(* Logix 5000 AddOnInstructionDefinition export SPEL_Above; software revision 30.01; part 7 of 9 *)

ADD_ON_INSTRUCTION SPEL_PointCoordGet   (* revision 1.2, vendor SEIKO EPSON CORP. *)
// Acquires the coordinate of the specified point.
VAR_OUTPUT
   InCycle : BOOL; {access Read Only, visible}
   Done : BOOL; {access Read Only, visible}
   Error : BOOL; {access Read Only, visible}
END_VAR
VAR_INPUT
   Start : BOOL; {access None, required}
   Point : INT; {access None, required}
   AxisNum : INT; {access None, required}
END_VAR
VAR_OUTPUT
   Value : REAL; {access Read Only, visible}
END_VAR
VAR_IN_OUT
   ExtInputs : AB:ETHERNET_MODULE_INT_128Bytes:I:0; {required}
   ExtOutputs : AB:ETHERNET_MODULE_INT_128Bytes:O:0; {required}
END_VAR
VAR_INPUT
   ErrCode1 : INT; {access None, visible}
   ErrCode2 : INT; {access None, visible}
END_VAR
VAR
   OneShotStart : BOOL; {access None}
   StartInit : BOOL; {access None}
   ExecGetPointCoord : SPEL_ExecCmd := (MaxTime := 3000); {access None}
   Coordinate_INTS : INT[2]; {access None}
   Coordinatex1000 : DINT; {access None}
END_VAR

ROUTINE Logic   (* ladder *)
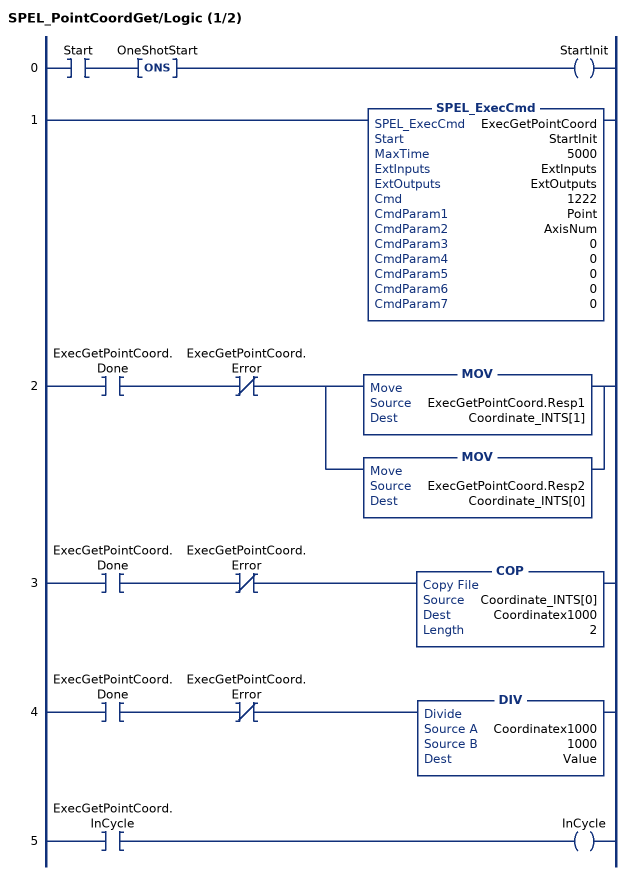
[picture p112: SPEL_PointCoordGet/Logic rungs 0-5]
   0: XIC(Start)ONS(OneShotStart)OTE(StartInit);
   1: SPEL_ExecCmd(ExecGetPointCoord,StartInit,5000,ExtInputs,ExtOutputs,1222,Point,AxisNum,0,0,0,0,0);
   2: XIC(ExecGetPointCoord.Done)XIO(ExecGetPointCoord.Error)[MOV(ExecGetPointCoord.Resp1,Coordinate_INTS[1]) ,MOV(ExecGetPointCoord.Resp2,Coordinate_INTS[0]) ];
   3: XIC(ExecGetPointCoord.Done)XIO(ExecGetPointCoord.Error)COP(Coordinate_INTS[0],Coordinatex1000,2);
   4: XIC(ExecGetPointCoord.Done)XIO(ExecGetPointCoord.Error)DIV(Coordinatex1000,1000,Value);
   5: XIC(ExecGetPointCoord.InCycle)OTE(InCycle);
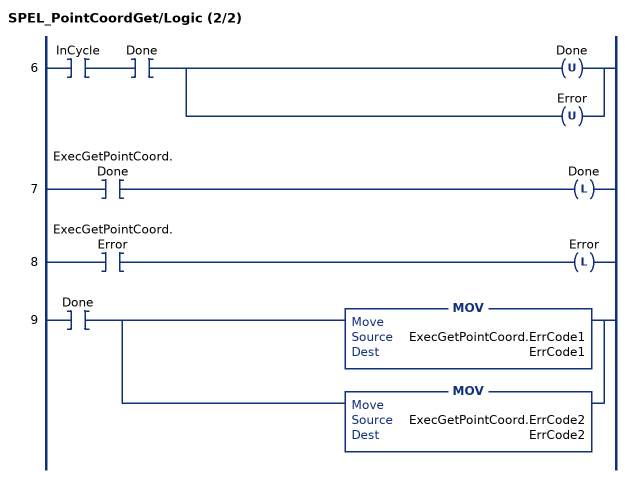
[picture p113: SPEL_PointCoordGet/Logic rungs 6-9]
   6: XIC(InCycle)XIC(Done)[OTU(Done) ,OTU(Error) ];
   7: XIC(ExecGetPointCoord.Done)OTL(Done);
   8: XIC(ExecGetPointCoord.Error)OTL(Error);
   9: XIC(Done)[MOV(ExecGetPointCoord.ErrCode1,ErrCode1) ,MOV(ExecGetPointCoord.ErrCode2,ErrCode2) ];
END_ROUTINE
END_ADD_ON_INSTRUCTION

ADD_ON_INSTRUCTION SPEL_PointCoordSet   (* revision 1.2, vendor SEIKO EPSON CORP. *)
// Sets the specified coordinate value to the coordinate of specified axis.
VAR_OUTPUT
   InCycle : BOOL; {access Read Only, visible}
   Done : BOOL; {access Read Only, visible}
   Error : BOOL; {access Read Only, visible}
END_VAR
VAR_INPUT
   Start : BOOL; {access None, required}
   Point : INT; {access None, required}
   AxisNum : INT; {access None, required}
   Value : REAL; {access None, required}
END_VAR
VAR_IN_OUT
   ExtInputs : AB:ETHERNET_MODULE_INT_128Bytes:I:0; {required}
   ExtOutputs : AB:ETHERNET_MODULE_INT_128Bytes:O:0; {required}
END_VAR
VAR_OUTPUT
   ErrCode1 : DINT; {access Read Only, visible}
   ErrCode2 : DINT; {access Read Only, visible}
END_VAR
VAR
   OneShotStart : BOOL; {access None}
   StartInit : BOOL; {access None}
   ExecSetPoint : SPEL_ExecCmd := (MaxTime := 3000); {access None}
   Value1000 : DINT; {access None}
   ValueCoord_INT : INT[2]; {access None}
END_VAR

ROUTINE Logic   (* ladder *)
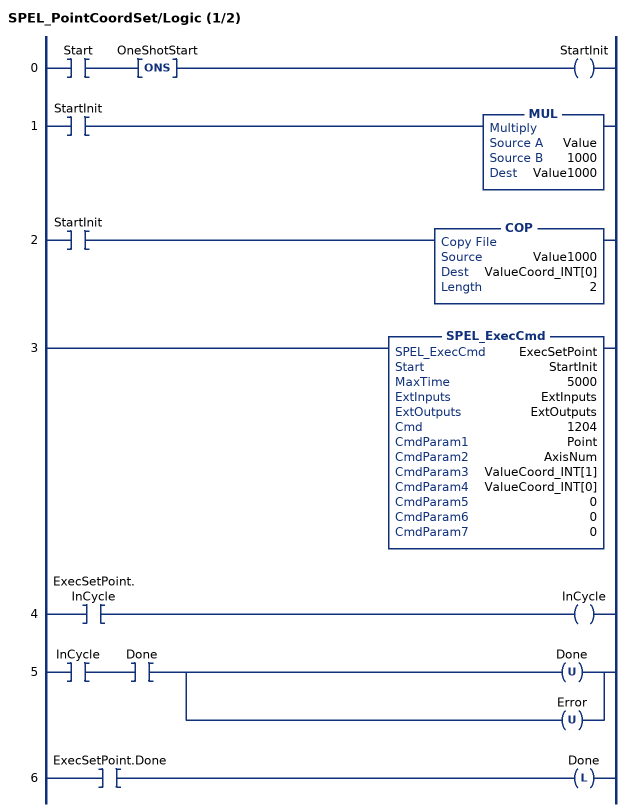
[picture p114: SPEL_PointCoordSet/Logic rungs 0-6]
   0: XIC(Start)ONS(OneShotStart)OTE(StartInit);
   1: XIC(StartInit)MUL(Value,1000,Value1000);
   2: XIC(StartInit)COP(Value1000,ValueCoord_INT[0],2);
   3: SPEL_ExecCmd(ExecSetPoint,StartInit,5000,ExtInputs,ExtOutputs,1204,Point,AxisNum,ValueCoord_INT[1],ValueCoord_INT[0],0,0,0);
   4: XIC(ExecSetPoint.InCycle)OTE(InCycle);
   5: XIC(InCycle)XIC(Done)[OTU(Done) ,OTU(Error) ];
   6: XIC(ExecSetPoint.Done)OTL(Done);
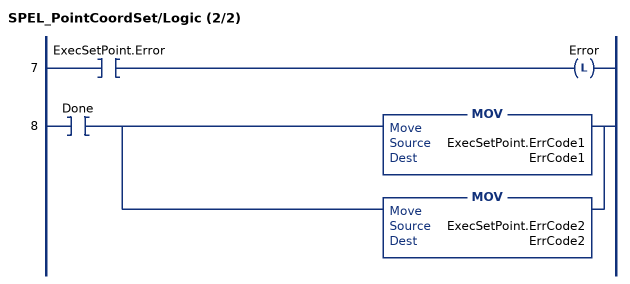
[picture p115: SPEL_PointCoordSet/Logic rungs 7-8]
   7: XIC(ExecSetPoint.Error)OTL(Error);
   8: XIC(Done)[MOV(ExecSetPoint.ErrCode1,ErrCode1) ,MOV(ExecSetPoint.ErrCode2,ErrCode2) ];
END_ROUTINE
END_ADD_ON_INSTRUCTION

ADD_ON_INSTRUCTION SPEL_PointSet   (* revision 1.2, vendor SEIKO EPSON CORP. *)
// Sets the specified coordinate value to the coordinate of specified axes.
VAR_OUTPUT
   InCycle : BOOL; {access Read Only, visible}
   Done : BOOL; {access Read Only, visible}
   Error : BOOL; {access Read Only, visible}
END_VAR
VAR_INPUT
   Start : BOOL; {access None, required}
   Point : INT; {access None, required}
   X : REAL; {access None, required}
   Y : REAL; {access None, required}
   Z : REAL; {access None, required}
   U : REAL; {access None, required}
   V : REAL; {access None, visible}
   W : REAL; {access None, visible}
END_VAR
VAR_IN_OUT
   ExtInputs : AB:ETHERNET_MODULE_INT_128Bytes:I:0; {required}
   ExtOutputs : AB:ETHERNET_MODULE_INT_128Bytes:O:0; {required}
END_VAR
VAR_OUTPUT
   ErrCode1 : INT; {access Read Only, visible}
   ErrCode2 : INT; {access Read Only, visible}
END_VAR
VAR
   OneShotInit : BOOL[32]; {access None}
   StartInit : BOOL[32]; {access None}
   ExecSetXY : SPEL_ExecCmd := (MaxTime := 3000); {access None}
   CoordinateX1000 : DINT; {access None}
   CoordinateX_INTS : INT[2]; {access None}
   CoordinateY_INTS : INT[2]; {access None}
   CoordinateY1000 : DINT; {access None}
   CoordinateZ1000 : DINT; {access None}
   CoordinateZ_INTS : INT[2]; {access None}
   CoordinateU1000 : DINT; {access None}
   CoordinateU_INTS : INT[2]; {access None}
   ExecSetZU : SPEL_ExecCmd := (MaxTime := 3000); {access None}
   CoordinateV1000 : DINT; {access None}
   CoordinateV_INTS : INT[2]; {access None}
   CoordinateW1000 : DINT; {access None}
   CoordinateW_INTS : INT[2]; {access None}
   ExecSetVW : SPEL_ExecCmd := (MaxTime := 3000); {access None}
END_VAR

ROUTINE Logic   (* ladder *)
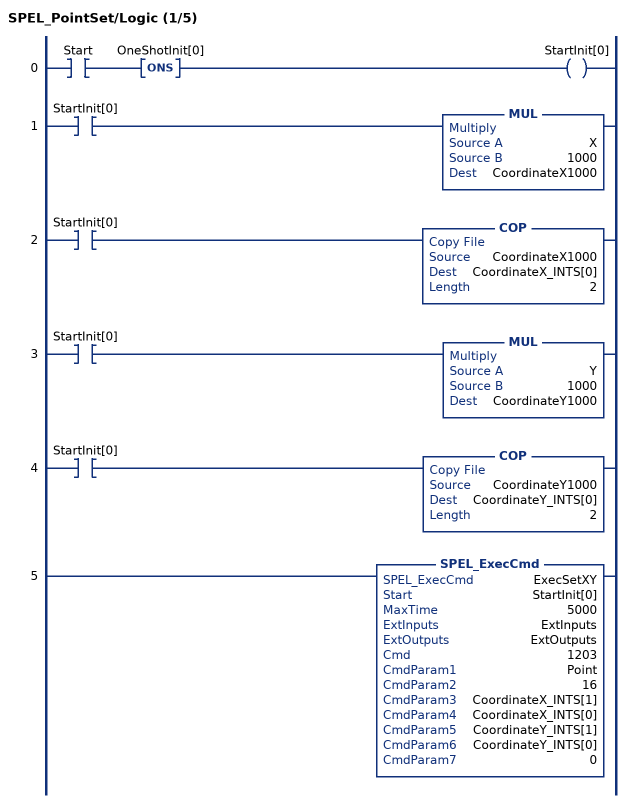
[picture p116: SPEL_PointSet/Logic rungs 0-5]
   0: XIC(Start)ONS(OneShotInit[0])OTE(StartInit[0]);
   1: XIC(StartInit[0])MUL(X,1000,CoordinateX1000);
   2: XIC(StartInit[0])COP(CoordinateX1000,CoordinateX_INTS[0],2);
   3: XIC(StartInit[0])MUL(Y,1000,CoordinateY1000);
   4: XIC(StartInit[0])COP(CoordinateY1000,CoordinateY_INTS[0],2);
   5: SPEL_ExecCmd(ExecSetXY,StartInit[0],5000,ExtInputs,ExtOutputs,1203,Point,16,CoordinateX_INTS[1],CoordinateX_INTS[0],CoordinateY_INTS[1],CoordinateY_INTS[0],0);
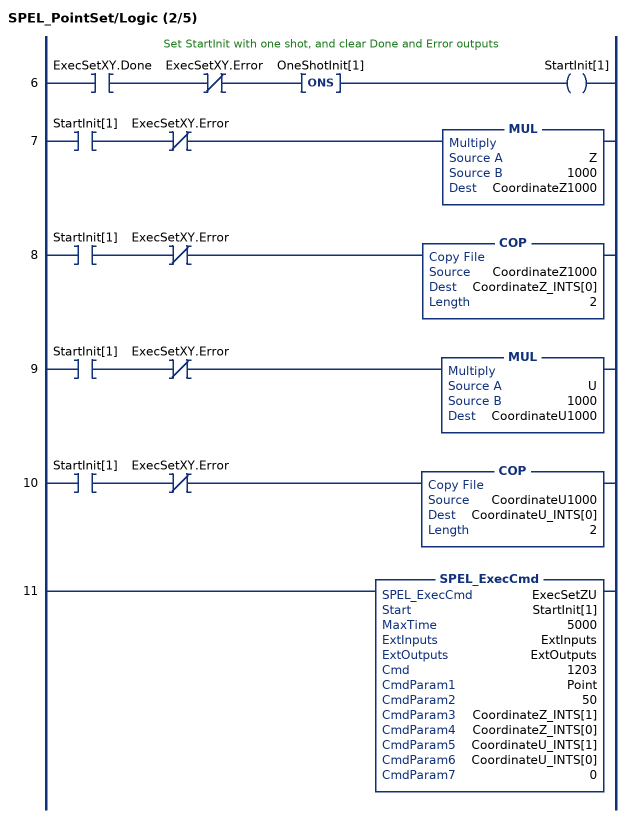
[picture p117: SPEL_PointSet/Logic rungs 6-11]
   // Set StartInit with one shot, and clear Done and Error outputs
   6: XIC(ExecSetXY.Done)XIO(ExecSetXY.Error)ONS(OneShotInit[1])OTE(StartInit[1]);
   7: XIC(StartInit[1])XIO(ExecSetXY.Error)MUL(Z,1000,CoordinateZ1000);
   8: XIC(StartInit[1])XIO(ExecSetXY.Error)COP(CoordinateZ1000,CoordinateZ_INTS[0],2);
   9: XIC(StartInit[1])XIO(ExecSetXY.Error)MUL(U,1000,CoordinateU1000);
   10: XIC(StartInit[1])XIO(ExecSetXY.Error)COP(CoordinateU1000,CoordinateU_INTS[0],2);
   11: SPEL_ExecCmd(ExecSetZU,StartInit[1],5000,ExtInputs,ExtOutputs,1203,Point,50,CoordinateZ_INTS[1],CoordinateZ_INTS[0],CoordinateU_INTS[1],CoordinateU_INTS[0],0);
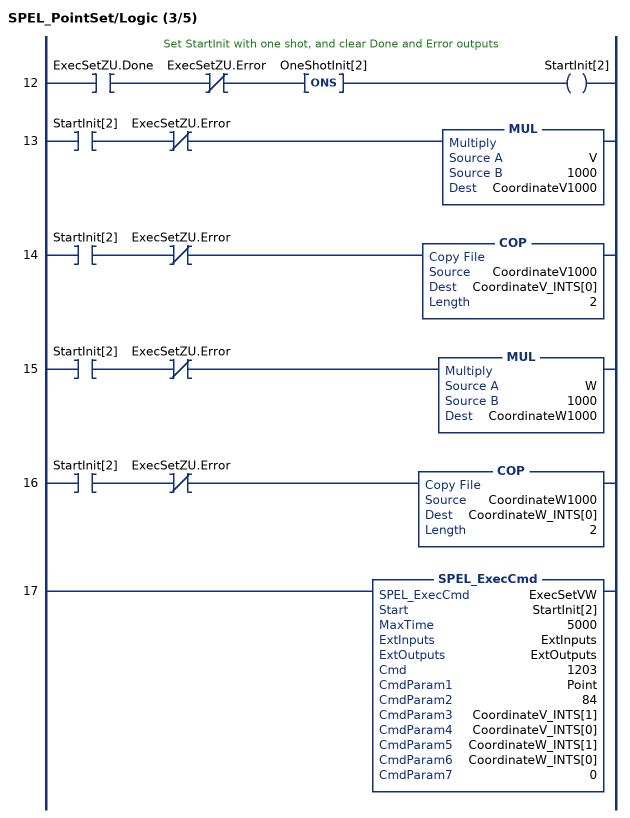
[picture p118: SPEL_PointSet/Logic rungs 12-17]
   // Set StartInit with one shot, and clear Done and Error outputs
   12: XIC(ExecSetZU.Done)XIO(ExecSetZU.Error)ONS(OneShotInit[2])OTE(StartInit[2]);
   13: XIC(StartInit[2])XIO(ExecSetZU.Error)MUL(V,1000,CoordinateV1000);
   14: XIC(StartInit[2])XIO(ExecSetZU.Error)COP(CoordinateV1000,CoordinateV_INTS[0],2);
   15: XIC(StartInit[2])XIO(ExecSetZU.Error)MUL(W,1000,CoordinateW1000);
   16: XIC(StartInit[2])XIO(ExecSetZU.Error)COP(CoordinateW1000,CoordinateW_INTS[0],2);
   17: SPEL_ExecCmd(ExecSetVW,StartInit[2],5000,ExtInputs,ExtOutputs,1203,Point,84,CoordinateV_INTS[1],CoordinateV_INTS[0],CoordinateW_INTS[1],CoordinateW_INTS[0],0);
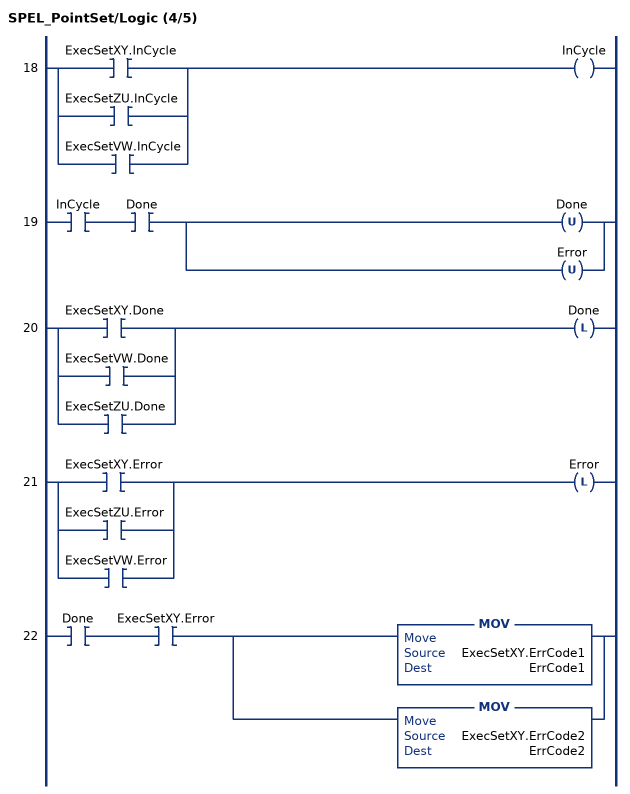
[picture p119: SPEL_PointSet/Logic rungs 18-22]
   18: [XIC(ExecSetXY.InCycle) ,XIC(ExecSetZU.InCycle) ,XIC(ExecSetVW.InCycle) ]OTE(InCycle);
   19: XIC(InCycle)XIC(Done)[OTU(Done) ,OTU(Error) ];
   20: [XIC(ExecSetXY.Done) ,XIC(ExecSetVW.Done) ,XIC(ExecSetZU.Done) ]OTL(Done);
   21: [XIC(ExecSetXY.Error) ,XIC(ExecSetZU.Error) ,XIC(ExecSetVW.Error) ]OTL(Error);
   22: XIC(Done)XIC(ExecSetXY.Error)[MOV(ExecSetXY.ErrCode1,ErrCode1) ,MOV(ExecSetXY.ErrCode2,ErrCode2) ];
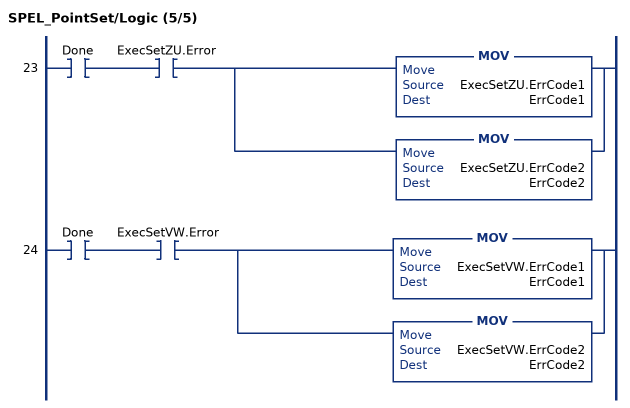
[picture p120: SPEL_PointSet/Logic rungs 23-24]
   23: XIC(Done)XIC(ExecSetZU.Error)[MOV(ExecSetZU.ErrCode1,ErrCode1) ,MOV(ExecSetZU.ErrCode2,ErrCode2) ];
   24: XIC(Done)XIC(ExecSetVW.Error)[MOV(ExecSetVW.ErrCode1,ErrCode1) ,MOV(ExecSetVW.ErrCode2,ErrCode2) ];
END_ROUTINE
END_ADD_ON_INSTRUCTION

ADD_ON_INSTRUCTION SPEL_PowerGet   (* revision 1.2, vendor SEIKO EPSON CORP. *)
// Gets the power control state.
VAR_INPUT
   Start : BOOL; {required}
END_VAR
VAR_OUTPUT
   InCycle : BOOL; {access Read Only, visible}
   Done : BOOL; {visible}
   Error : BOOL; {visible}
END_VAR
VAR_IN_OUT
   ExtInputs : AB:ETHERNET_MODULE_INT_128Bytes:I:0; {required}
   ExtOutputs : AB:ETHERNET_MODULE_INT_128Bytes:O:0; {required}
END_VAR
VAR_OUTPUT
   ErrCode1 : INT; {access Read Only, visible}
   ErrCode2 : INT; {access Read Only, visible}
   Status : INT; {visible}
END_VAR
VAR
   ExecPower : SPEL_ExecCmd := (MaxTime := 3000); {access None}
   ExecTimeout : DINT; {access None}
END_VAR

ROUTINE Logic   (* ladder *)
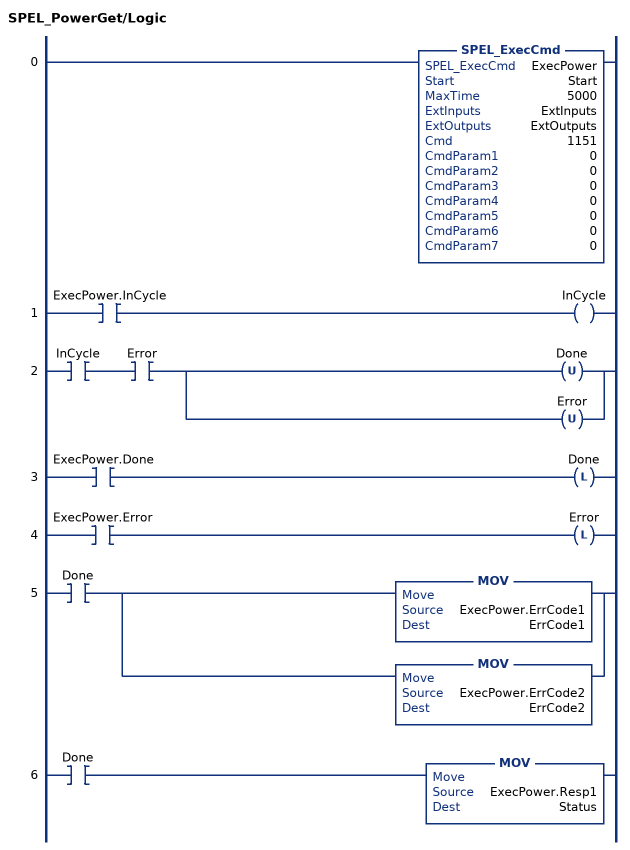
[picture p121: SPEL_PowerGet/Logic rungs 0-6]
   0: SPEL_ExecCmd(ExecPower,Start,5000,ExtInputs,ExtOutputs,1151,0,0,0,0,0,0,0);
   1: XIC(ExecPower.InCycle)OTE(InCycle);
   2: XIC(InCycle)XIC(Error)[OTU(Done) ,OTU(Error) ];
   3: XIC(ExecPower.Done)OTL(Done);
   4: XIC(ExecPower.Error)OTL(Error);
   5: XIC(Done)[MOV(ExecPower.ErrCode1,ErrCode1) ,MOV(ExecPower.ErrCode2,ErrCode2) ];
   6: XIC(Done)MOV(ExecPower.Resp1,Status);
END_ROUTINE
END_ADD_ON_INSTRUCTION

ADD_ON_INSTRUCTION SPEL_PowerHigh   (* revision 1.0, vendor SEIKO EPSON CORP. *)
// Sets the power level of robot to high.
VAR_OUTPUT
   InCycle : BOOL; {access Read Only, visible}
   Done : BOOL; {access Read Only, visible}
   Error : BOOL; {access Read Only, visible}
END_VAR
VAR_INPUT
   Start : BOOL; {required}
END_VAR
VAR_IN_OUT
   ExtInputs : AB:ETHERNET_MODULE_INT_128Bytes:I:0; {required}
   ExtOutputs : AB:ETHERNET_MODULE_INT_128Bytes:O:0; {required}
END_VAR
VAR_OUTPUT
   ErrCode1 : INT; {access Read Only, visible}
   ErrCode2 : INT; {access Read Only, visible}
END_VAR
VAR
   ExecPowerHigh : SPEL_ExecCmd := (MaxTime := 3000); {access None}
        .INCYCLE   // ExecInCycle
        .DONE   // ExecDone
        .ERROR   // ExecError
   OneShotStart : BOOL; {access None}
   StartCoil : BOOL; {access None}
   ExecTimeout : DINT; {access None}
END_VAR

ROUTINE Logic   (* ladder *)
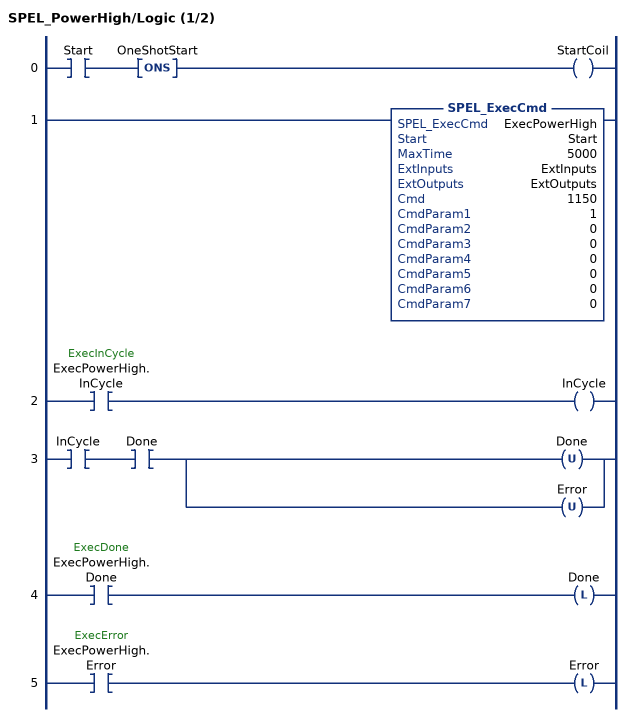
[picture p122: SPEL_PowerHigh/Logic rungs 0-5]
   0: XIC(Start)ONS(OneShotStart)OTE(StartCoil);
   1: SPEL_ExecCmd(ExecPowerHigh,Start,5000,ExtInputs,ExtOutputs,1150,1,0,0,0,0,0,0);
   2: XIC(ExecPowerHigh.InCycle)OTE(InCycle);
   3: XIC(InCycle)XIC(Done)[OTU(Done) ,OTU(Error) ];
   4: XIC(ExecPowerHigh.Done)OTL(Done);
   5: XIC(ExecPowerHigh.Error)OTL(Error);
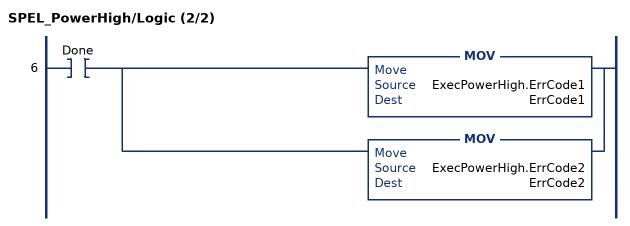
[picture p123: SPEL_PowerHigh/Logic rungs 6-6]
   6: XIC(Done)[MOV(ExecPowerHigh.ErrCode1,ErrCode1) ,MOV(ExecPowerHigh.ErrCode2,ErrCode2) ];
END_ROUTINE
END_ADD_ON_INSTRUCTION

ADD_ON_INSTRUCTION SPEL_PowerLow   (* revision 1.0, vendor SEIKO EPSON CORP. *)
// Sets the power level of robot to low.
VAR_OUTPUT
   InCycle : BOOL; {access Read Only, visible}
   Done : BOOL; {access Read Only, visible}
   Error : BOOL; {access Read Only, visible}
END_VAR
VAR_INPUT
   Start : BOOL; {required}
END_VAR
VAR_IN_OUT
   ExtInputs : AB:ETHERNET_MODULE_INT_128Bytes:I:0; {required}
   ExtOutputs : AB:ETHERNET_MODULE_INT_128Bytes:O:0; {required}
END_VAR
VAR_OUTPUT
   ErrCode1 : INT; {access Read Only, visible}
   ErrCode2 : INT; {access Read Only, visible}
END_VAR
VAR
   ExecPowerLow : SPEL_ExecCmd := (MaxTime := 3000); {access None}
        .INCYCLE   // ExecInCycle
        .DONE   // ExecDone
        .ERROR   // ExecError
   OneShotStart : BOOL; {access None}
   StartCoil : BOOL; {access None}
   ExecTimeout : DINT; {access None}
END_VAR

ROUTINE Logic   (* ladder *)
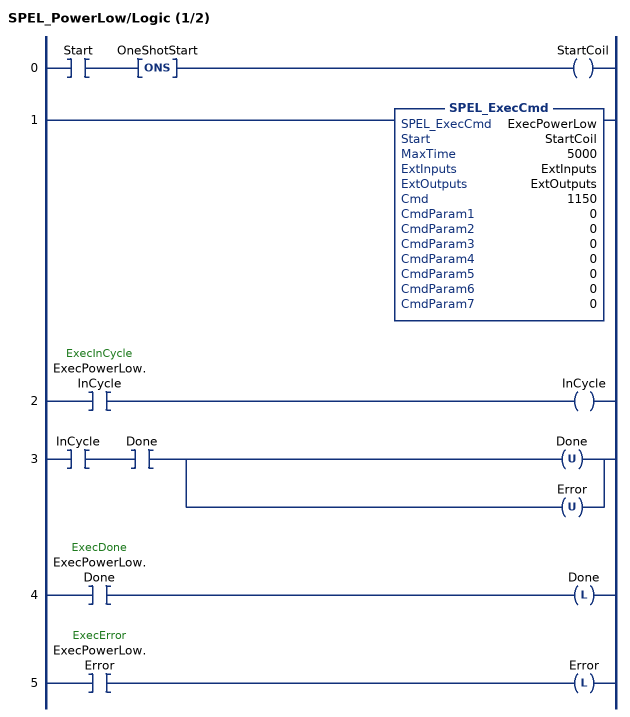
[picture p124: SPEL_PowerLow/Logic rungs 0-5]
   0: XIC(Start)ONS(OneShotStart)OTE(StartCoil);
   1: SPEL_ExecCmd(ExecPowerLow,StartCoil,5000,ExtInputs,ExtOutputs,1150,0,0,0,0,0,0,0);
   2: XIC(ExecPowerLow.InCycle)OTE(InCycle);
   3: XIC(InCycle)XIC(Done)[OTU(Done) ,OTU(Error) ];
   4: XIC(ExecPowerLow.Done)OTL(Done);
   5: XIC(ExecPowerLow.Error)OTL(Error);
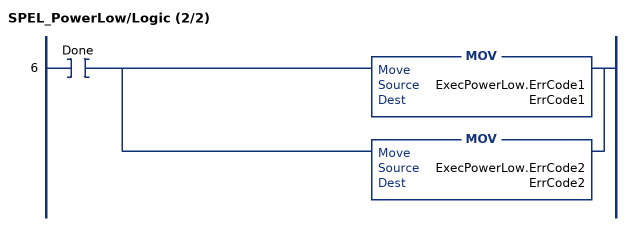
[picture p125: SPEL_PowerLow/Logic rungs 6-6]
   6: XIC(Done)[MOV(ExecPowerLow.ErrCode1,ErrCode1) ,MOV(ExecPowerLow.ErrCode2,ErrCode2) ];
END_ROUTINE
END_ADD_ON_INSTRUCTION

ADD_ON_INSTRUCTION SPEL_Reset   (* revision 1.0, vendor SEIKO EPSON CORP. *)
// Resets the robot controller to an initialized state.
VAR_INPUT
   Start : BOOL; {required}
END_VAR
VAR_IN_OUT
   ExtInputs : AB:ETHERNET_MODULE_INT_128Bytes:I:0; {required}
   ExtOutputs : AB:ETHERNET_MODULE_INT_128Bytes:O:0; {required}
END_VAR
VAR_OUTPUT
   ErrCode1 : INT; {access Read Only, visible}
   ErrCode2 : INT; {access Read Only, visible}
   InCycle : BOOL; {access Read Only, visible}
   Done : BOOL; {access Read Only, visible}
   Error : BOOL; {access Read Only, visible}
END_VAR
VAR
   ExecReset : SPEL_ExecCmd := (MaxTime := 3000); {access None}   // Execute controller reset
   OneShotStart : BOOL; {access None}
   StartCoil : BOOL; {access None}
   ExecTimeout : DINT; {access None}
END_VAR

ROUTINE Logic   (* ladder *)
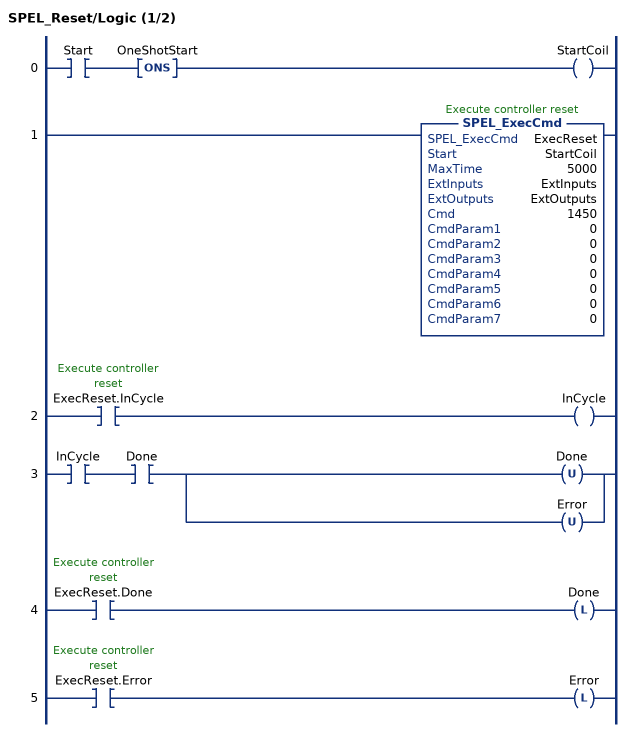
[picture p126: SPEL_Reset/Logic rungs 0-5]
   0: XIC(Start)ONS(OneShotStart)OTE(StartCoil);
   1: SPEL_ExecCmd(ExecReset,StartCoil,5000,ExtInputs,ExtOutputs,1450,0,0,0,0,0,0,0);
   2: XIC(ExecReset.InCycle)OTE(InCycle);
   3: XIC(InCycle)XIC(Done)[OTU(Done) ,OTU(Error) ];
   4: XIC(ExecReset.Done)OTL(Done);
   5: XIC(ExecReset.Error)OTL(Error);
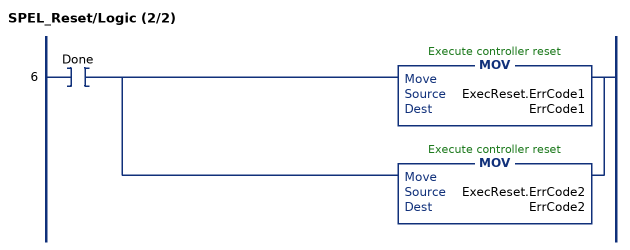
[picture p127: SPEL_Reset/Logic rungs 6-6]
   6: XIC(Done)[MOV(ExecReset.ErrCode1,ErrCode1) ,MOV(ExecReset.ErrCode2,ErrCode2) ];
END_ROUTINE
END_ADD_ON_INSTRUCTION

ADD_ON_INSTRUCTION SPEL_Righty   (* revision 1.0, vendor SEIKO EPSON CORP. *)
// Sets the hand orientation of the specified point to Righty.
VAR_OUTPUT
   InCycle : BOOL; {access Read Only, visible}
   Done : BOOL; {access Read Only, visible}
   Error : BOOL; {access Read Only, visible}
END_VAR
VAR_INPUT
   Start : BOOL; {required}
   Point : INT; {required}
END_VAR
VAR_IN_OUT
   ExtInputs : AB:ETHERNET_MODULE_INT_128Bytes:I:0; {required}
   ExtOutputs : AB:ETHERNET_MODULE_INT_128Bytes:O:0; {required}
END_VAR
VAR_OUTPUT
   ErrCode1 : INT; {access Read Only, visible}
   ErrCode2 : INT; {access Read Only, visible}
END_VAR
VAR
   ExecRighty : SPEL_ExecCmd := (MaxTime := 3000); {access None}
   OneShotStart : BOOL; {access None}
   StartCoil : BOOL; {access None}
   ExecTimeout : DINT; {access None}
END_VAR

ROUTINE Logic   (* ladder *)
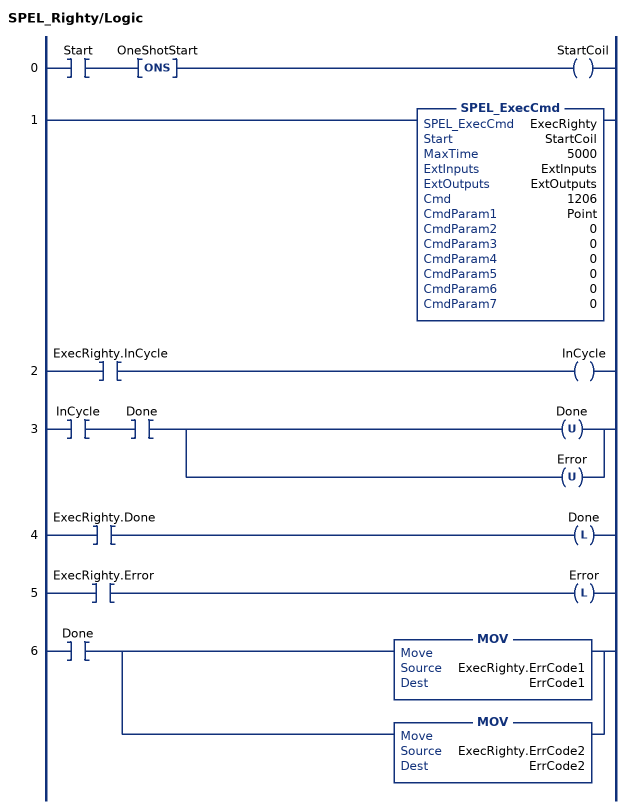
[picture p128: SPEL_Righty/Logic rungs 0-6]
   0: XIC(Start)ONS(OneShotStart)OTE(StartCoil);
   1: SPEL_ExecCmd(ExecRighty,StartCoil,5000,ExtInputs,ExtOutputs,1206,Point,0,0,0,0,0,0);
   2: XIC(ExecRighty.InCycle)OTE(InCycle);
   3: XIC(InCycle)XIC(Done)[OTU(Done) ,OTU(Error) ];
   4: XIC(ExecRighty.Done)OTL(Done);
   5: XIC(ExecRighty.Error)OTL(Error);
   6: XIC(Done)[MOV(ExecRighty.ErrCode1,ErrCode1) ,MOV(ExecRighty.ErrCode2,ErrCode2) ];
END_ROUTINE
END_ADD_ON_INSTRUCTION

ADD_ON_INSTRUCTION SPEL_SavePoints   (* revision 1.0, vendor SEIKO EPSON CORP. *)
// Saves the current point setting to the point file.
VAR_OUTPUT
   InCycle : BOOL; {access Read Only, visible}
   Done : BOOL; {access Read Only, visible}
   Error : BOOL; {access Read Only, visible}
END_VAR
VAR_INPUT
   Start : BOOL; {required}
END_VAR
VAR_IN_OUT
   ExtInputs : AB:ETHERNET_MODULE_INT_128Bytes:I:0; {required}
   ExtOutputs : AB:ETHERNET_MODULE_INT_128Bytes:O:0; {required}
END_VAR
VAR_OUTPUT
   ErrCode1 : INT; {access Read Only, visible}
   ErrCode2 : INT; {access Read Only, visible}
END_VAR
VAR
   ExecSaveP : SPEL_ExecCmd := (MaxTime := 3000); {access None}
   OneShotStart : BOOL; {access None}
   StartCoil : BOOL; {access None}
   ExecTimeout : DINT; {access None}
END_VAR

ROUTINE Logic   (* ladder *)
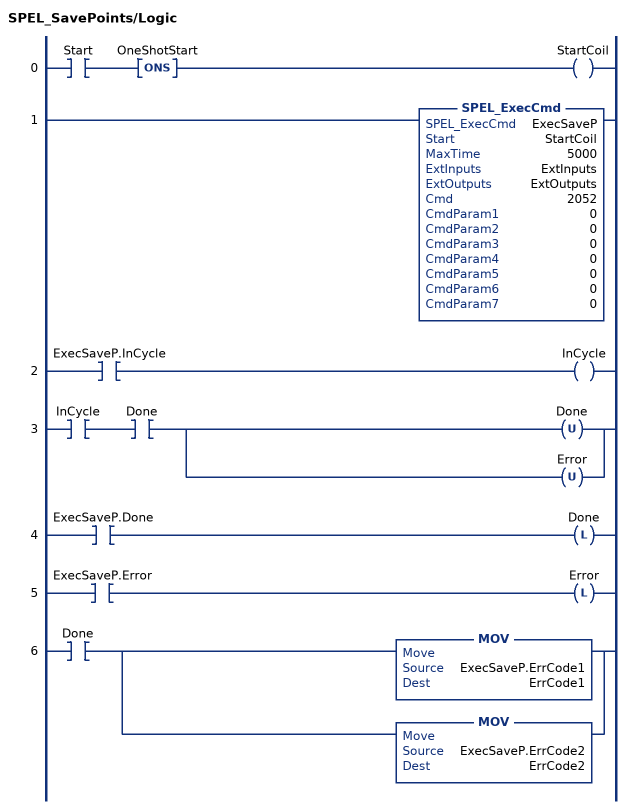
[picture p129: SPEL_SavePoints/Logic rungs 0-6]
   0: XIC(Start)ONS(OneShotStart)OTE(StartCoil);
   1: SPEL_ExecCmd(ExecSaveP,StartCoil,5000,ExtInputs,ExtOutputs,2052,0,0,0,0,0,0,0);
   2: XIC(ExecSaveP.InCycle)OTE(InCycle);
   3: XIC(InCycle)XIC(Done)[OTU(Done) ,OTU(Error) ];
   4: XIC(ExecSaveP.Done)OTL(Done);
   5: XIC(ExecSaveP.Error)OTL(Error);
   6: XIC(Done)[MOV(ExecSaveP.ErrCode1,ErrCode1) ,MOV(ExecSaveP.ErrCode2,ErrCode2) ];
END_ROUTINE
END_ADD_ON_INSTRUCTION
